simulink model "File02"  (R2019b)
settings: Solver=FixedStepDiscrete  StartTime=0.0  StopTime=10.0  FixedStep=1  RelTol=1e-3
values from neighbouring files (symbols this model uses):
  A = [0.5 0;0 2]    [File02_dati.m]
  B = [2;1]    [File02_dati.m]
  C = [1 2]    [File02_dati.m]
  D = 0    [File02_dati.m]
  Xzero = [1;2]    [File02_dati.m]

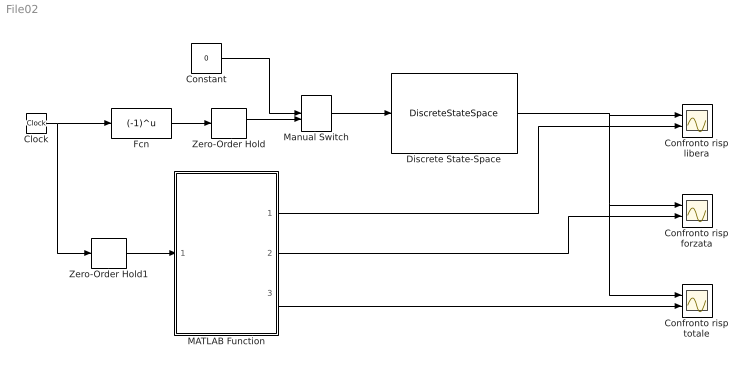
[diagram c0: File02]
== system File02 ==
  Clock : Clock
  Confronto risp forzata : Scope  NumInputPorts=2
  Confronto risp libera : Scope  NumInputPorts=2
  Confronto risp totale : Scope  NumInputPorts=2
  Constant : Constant  Value=0
  Discrete State-Space : DiscreteStateSpace  A=A  B=B  C=C  D=D  InitialCondition=Xzero  SampleTime=-1
  Fcn : Fcn  Expr=(-1)^u
  MATLAB Function : MATLAB Function  TreatAsAtomicUnit=on
  Manual Switch : ManualSwitch  CurrentSetting=0
  Zero-Order Hold : ZeroOrderHold
  Zero-Order Hold1 : ZeroOrderHold
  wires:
  Clock/1 -> Zero-Order Hold1/1, Fcn/1
  Fcn/1 -> Zero-Order Hold/1
  Manual Switch/1 -> Discrete State-Space/1
  Zero-Order Hold/1 -> Manual Switch/2
  Constant/1 -> Manual Switch/1
  Discrete State-Space/1 -> Confronto risp totale/1, Confronto risp forzata/1, Confronto risp libera/1
  MATLAB Function/1(yl) -> Confronto risp libera/2
  Zero-Order Hold1/1 -> MATLAB Function/1(k)
  MATLAB Function/2(yf) -> Confronto risp forzata/2
  MATLAB Function/3(ytot) -> Confronto risp totale/2

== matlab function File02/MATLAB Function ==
function [yl,yf,ytot] = fcn(k)

yl=(0.5)^k+4*2^k;
yf=-2*(-1)^k+1.333*(0.5)^k+0.6666*(2)^k;
ytot = yl+yf;
